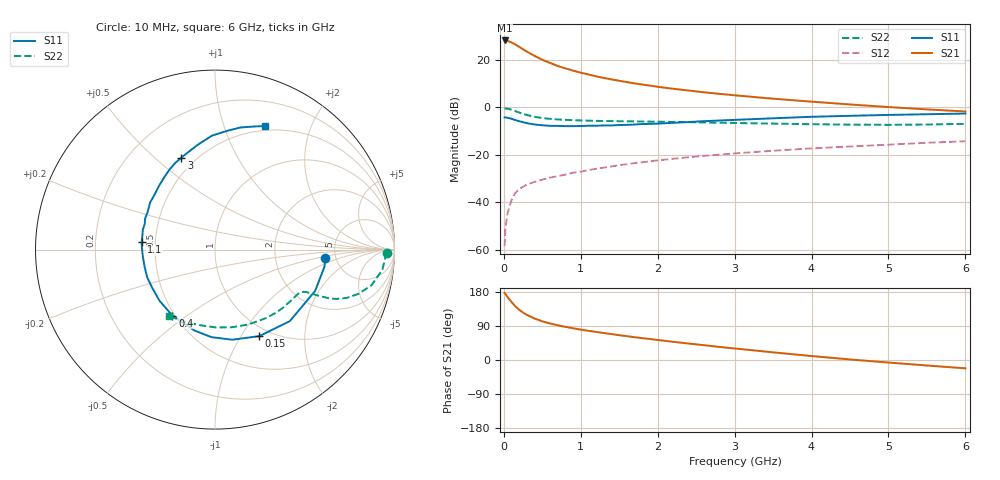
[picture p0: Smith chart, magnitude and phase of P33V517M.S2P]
! SIEMENS Small Signal Semiconductors
! BFP181
! Si NPN RF Bipolar Junction Transistor in SOT143
! VCE = 3.5 V  IC = 17 mA
! Common Emitter S-Parameters:  March  1996
# GHz  S  MA  R  50
!  f  S11  S21  S12  S22
! GHz  MAG  ANG  MAG  ANG  MAG  ANG  MAG  ANG
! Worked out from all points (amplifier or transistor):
!   36 points, 10 MHz to 6 GHz, reference 50 ohm
!   highest |S21| = 28.2 dB at 10 MHz (marker M1)
!   |S21| within 3 dB of that: start of sweep to 214.6 MHz
!   unconditionally stable (mu >= 1): 679.4 MHz to end of sweep
!   at 250 MHz: K = 0.51, MSG = 28.9 dB, |S12| = -33.4 dB
!   at 1.4 GHz: K = 1.26, MAG = 15.2 dB, |S12| = -24.9 dB
!   at 6 GHz: K = 1.03, MAG = 5.3 dB, |S12| = -14.2 dB
!   S11 on the Smith chart (normalised r, x): 10 MHz: 4.10, -0.65; 150 MHz: 0.88, -1.21; 400 MHz: 0.49, -0.44; 1.1 GHz: 0.42, +0.04; 3 GHz: 0.42, +0.61; 6 GHz: 0.45, +1.38
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0.01  0.6158 -4.6  25.66 176.8  0.0012 85.5  0.9558 -1.0
0.02  0.6173 -8.9  25.61 174.4  0.0028 83.4  0.9499 -2.6
0.05  0.6034 -22.5  25.16 165.8  0.0061 83.0  0.9395 -6.9
0.1  0.5767 -43.7  23.21 153.0  0.0112 70.5  0.8935 -12.9
0.15  0.5416 -62.9  21.06 141.6  0.0159 64.8  0.8357 -17.2
0.2  0.5113 -79.1  18.82 132.4  0.0192 59.9  0.7802 -20.2
0.25  0.4882 -92.3  16.68 125.0  0.0214 57.5  0.7305 -22.1
0.3  0.4653 -104.1  14.93 119.1  0.0239 55.1  0.6925 -23.1
0.4  0.4373 -122.9  12.12 109.3  0.027 53.0  0.6342 -24.0
0.5  0.4206 -137.3  10.06 102.1  0.0302 51.4  0.5973 -24.4
0.6  0.4096 -148.9  8.654 96.5  0.0333 53.1  0.5742 -24.7
0.7  0.4082 -157.9  7.455 91.7  0.0357 52.7  0.5575 -25.0
0.9  0.4036 -173.0  5.953 83.8  0.0421 54.1  0.5379 -26.1
1.1  0.4113 174.3  4.932 76.9  0.0479 54.8  0.5255 -27.8
1.3  0.4171 164.5  4.164 71.1  0.0541 54.6  0.5186 -30.1
1.6  0.429 151.5  3.408 62.9  0.0638 54.5  0.5104 -33.7
2.2  0.4733 131.1  2.468 48.0  0.083 52.0  0.4945 -42.6
3  0.546 110.0  1.798 30.4  0.1074 46.8  0.4692 -56.5
3.5  0.5898 99.8  1.526 20.2  0.1224 43.3  0.4562 -66.4
4.5  0.6654 84.1  1.154 1.4  0.1505 35.1  0.4341 -89.1
5.5  0.7181 72.7  0.908 -14.5  0.18 27.5  0.4367 -112.9
6  0.7425 68.0  0.821 -22.0  0.194 23.3  0.4505 -124.9
